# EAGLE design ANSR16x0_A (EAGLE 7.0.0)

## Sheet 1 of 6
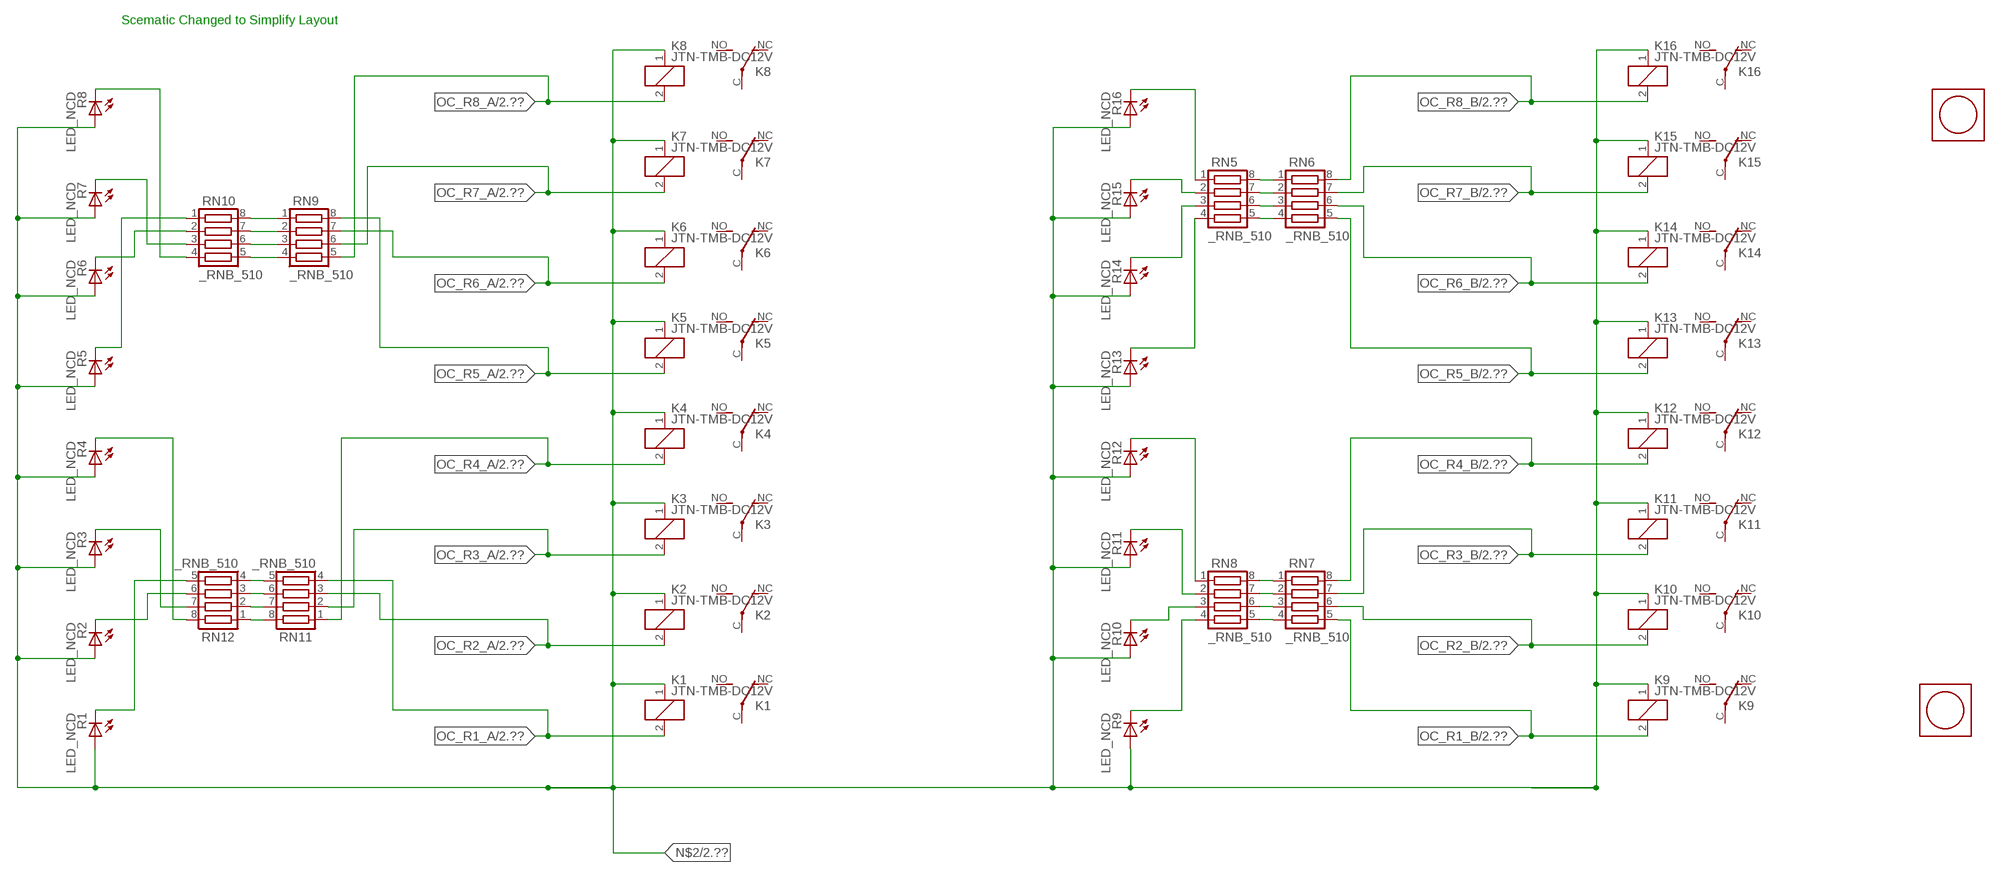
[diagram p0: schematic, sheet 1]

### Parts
K1  JTN-TMB-DC12V  [JT-TMB]
K2  JTN-TMB-DC12V  [JT-TMB]
K3  JTN-TMB-DC12V  [JT-TMB]
K4  JTN-TMB-DC12V  [JT-TMB]
K5  JTN-TMB-DC12V  [JT-TMB]
K6  JTN-TMB-DC12V  [JT-TMB]
K7  JTN-TMB-DC12V  [JT-TMB]
K8  JTN-TMB-DC12V  [JT-TMB]
K9  JTN-TMB-DC12V  [JT-TMB]
K10  JTN-TMB-DC12V  [JT-TMB]
K11  JTN-TMB-DC12V  [JT-TMB]
K12  JTN-TMB-DC12V  [JT-TMB]
K13  JTN-TMB-DC12V  [JT-TMB]
K14  JTN-TMB-DC12V  [JT-TMB]
K15  JTN-TMB-DC12V  [JT-TMB]
K16  JTN-TMB-DC12V  [JT-TMB]
R1  LED_NCD  [CHIPLED_0603]
R2  LED_NCD  [CHIPLED_0603]
R3  LED_NCD  [CHIPLED_0603]
R4  LED_NCD  [CHIPLED_0603]
R5  LED_NCD  [CHIPLED_0603]
R6  LED_NCD  [CHIPLED_0603]
R7  LED_NCD  [CHIPLED_0603]
R8  LED_NCD  [CHIPLED_0603]
R9  LED_NCD  [CHIPLED_0603]
R10  LED_NCD  [CHIPLED_0603]
R11  LED_NCD  [CHIPLED_0603]
R12  LED_NCD  [CHIPLED_0603]
R13  LED_NCD  [CHIPLED_0603]
R14  LED_NCD  [CHIPLED_0603]
R15  LED_NCD  [CHIPLED_0603]
R16  LED_NCD  [CHIPLED_0603]
RN5  _RNB_510  [RNB]
RN6  _RNB_510  [RNB]
RN7  _RNB_510  [RNB]
RN8  _RNB_510  [RNB]
RN9  _RNB_510  [RNB]
RN10  _RNB_510  [RNB]
RN11  _RNB_510  [RNB]
RN12  _RNB_510  [RNB]
U$1  PCB_MOUNTING_HOLE  [PCB_MOUNTING_HOLE]
U$3  PCB_MOUNTING_HOLE  [PCB_MOUNTING_HOLE]

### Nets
N$2: K1.1(C1) K2.1(C1) K3.1(C1) K4.1(C1) K5.1(C1) K6.1(C1) K7.1(C1) K8.1(C1) K9.1(C1) K10.1(C1) K11.1(C1) K12.1(C1) K13.1(C1) K14.1(C1) K15.1(C1) K16.1(C1) R1.A R2.A R3.A R4.A R5.A R6.A R7.A R8.A R9.A R10.A R11.A R12.A R13.A R14.A R15.A R16.A ; also sheet 2
N$441: R16.C RN5.1
N$442: RN7.2 RN8.7
N$443: RN7.3 RN8.6
N$444: RN7.4 RN8.5
N$445: R15.C RN5.2
N$447: R13.C RN5.4
N$448: RN5.5 RN6.4
N$449: RN7.1 RN8.8
N$450: R12.C RN8.1
N$451: RN5.6 RN6.3
N$452: R11.C RN8.2
N$453: RN5.7 RN6.2
N$454: RN5.8 RN6.1
N$458: R14.C RN5.3
N$459: R10.C RN8.3
N$463: RN11.5 RN12.4
N$470: R9.C RN8.4
N$473: R1.C RN12.5
N$474: RN11.6 RN12.3
N$475: R2.C RN12.6
N$476: R3.C RN12.7
N$477: RN9.4 RN10.5
N$478: RN9.3 RN10.6
N$479: RN9.2 RN10.7
N$480: RN9.1 RN10.8
N$481: RN11.7 RN12.2
N$482: R5.C RN10.1
N$483: R4.C RN12.8
N$484: R7.C RN10.3
N$485: R8.C RN10.4
N$486: R6.C RN10.2
N$500: RN11.8 RN12.1
OC_R1_A: K1.2(C2) RN11.4 ; also sheet 2
OC_R1_B: K9.2(C2) RN7.5 ; also sheet 2
OC_R2_A: K2.2(C2) RN11.3 ; also sheet 2
OC_R2_B: K10.2(C2) RN7.6 ; also sheet 2
OC_R3_A: K3.2(C2) RN11.2 ; also sheet 2
OC_R3_B: K11.2(C2) RN7.7 ; also sheet 2
OC_R4_A: K4.2(C2) RN11.1 ; also sheet 2
OC_R4_B: K12.2(C2) RN7.8 ; also sheet 2
OC_R5_A: K5.2(C2) RN9.8 ; also sheet 2
OC_R5_B: K13.2(C2) RN6.5 ; also sheet 2
OC_R6_A: K6.2(C2) RN9.7 ; also sheet 2
OC_R6_B: K14.2(C2) RN6.6 ; also sheet 2
OC_R7_A: K7.2(C2) RN9.6 ; also sheet 2
OC_R7_B: K15.2(C2) RN6.7 ; also sheet 2
OC_R8_A: K8.2(C2) RN9.5 ; also sheet 2
OC_R8_B: K16.2(C2) RN6.8 ; also sheet 2
Unconnected: K1.C(COM) K1.NC K1.NO K2.C(COM) K2.NC K2.NO K3.C(COM) K3.NC K3.NO K4.C(COM) K4.NC K4.NO K5.C(COM) K5.NC K5.NO K6.C(COM) K6.NC K6.NO K7.C(COM) K7.NC K7.NO K8.C(COM) K8.NC K8.NO K9.C(COM) K9.NC K9.NO K10.C(COM) K10.NC K10.NO K11.C(COM) K11.NC K11.NO K12.C(COM) K12.NC K12.NO K13.C(COM) K13.NC K13.NO K14.C(COM) K14.NC K14.NO K15.C(COM) K15.NC K15.NO K16.C(COM) K16.NC K16.NO

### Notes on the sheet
- Scematic Changed to Simplify Layout

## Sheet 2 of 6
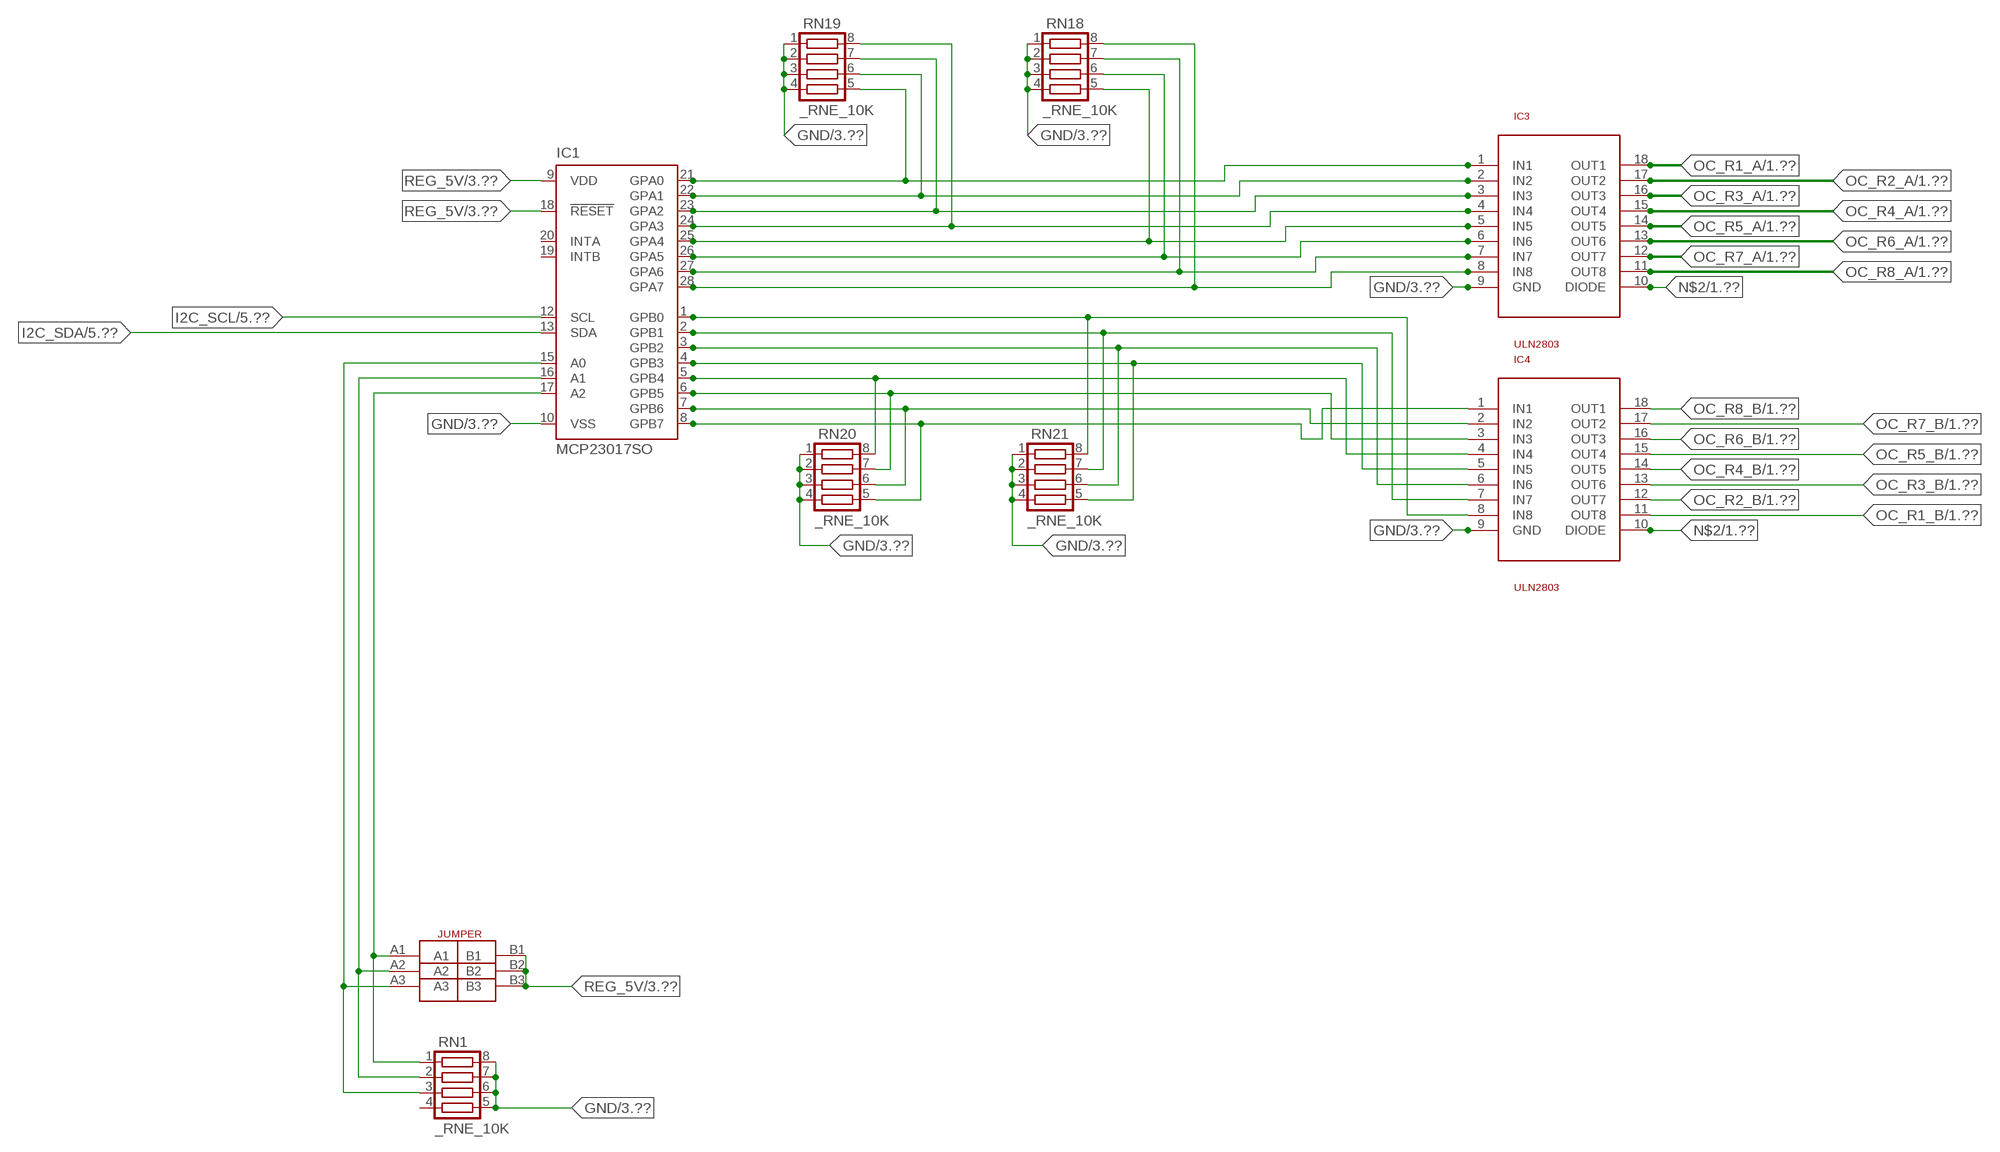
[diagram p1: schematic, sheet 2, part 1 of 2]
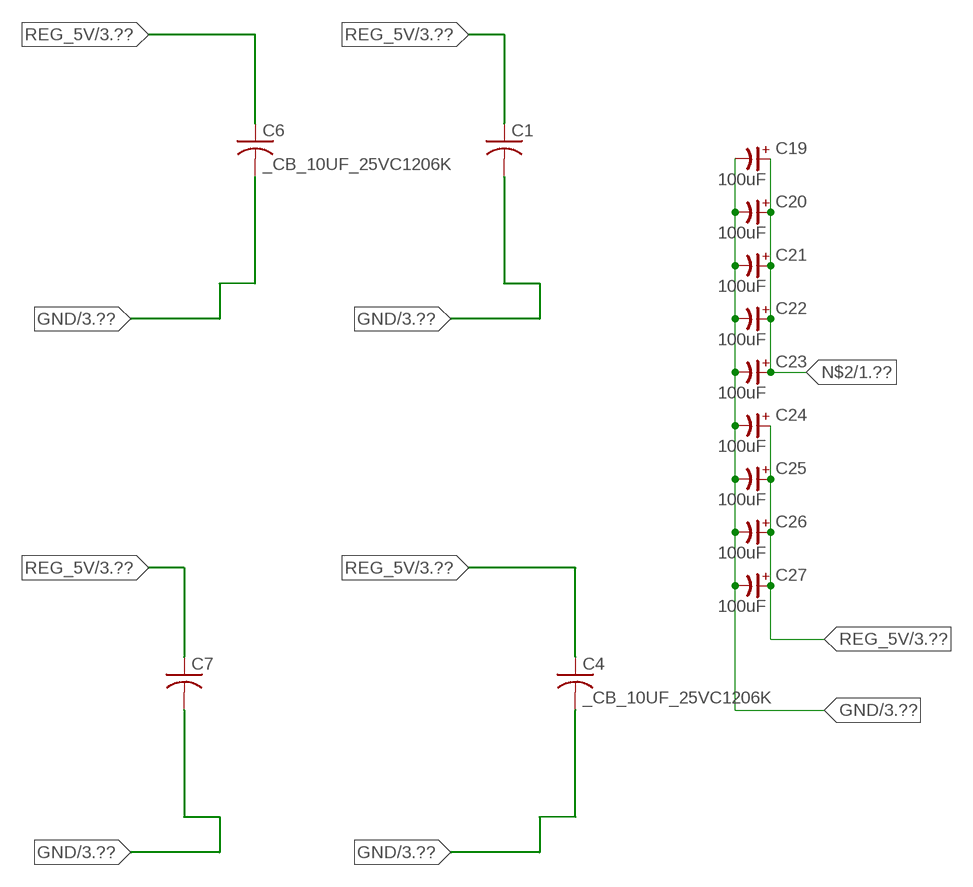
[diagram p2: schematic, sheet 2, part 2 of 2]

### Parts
C1  _CA_.10UF_50VC1206K  [_CA_.1UF_50V]
C4  _CB_10UF_25VC1206K  [_CB_10UF_25V]
C6  _CB_10UF_25VC1206K  [_CB_10UF_25V]
C7  _CA_.10UF_50VC1206K  [_CA_.1UF_50V]
C19  100uF  CP-E-025X060  [E-025X060]
C20  100uF  CP-E-025X060  [E-025X060]
C21  100uF  CP-E-025X060  [E-025X060]
C22  100uF  CP-E-025X060  [E-025X060]
C23  100uF  CP-E-025X060  [E-025X060]
C24  100uF  CP-E-025X060  [E-025X060]
C25  100uF  CP-E-025X060  [E-025X060]
C26  100uF  CP-E-025X060  [E-025X060]
C27  100uF  CP-E-025X060  [E-025X060]
IC1  MCP23017SO  [SO28W]
IC3  ULN2803  [SO18L]
IC4  ULN2803  [SO18L]
JP1  JUMPER_3X2  [JUMPER_3X2]
RN1  _RNE_10K  [RNE]
RN18  _RNE_10K  [RNE]
RN19  _RNE_10K  [RNE]
RN20  _RNE_10K  [RNE]
RN21  _RNE_10K  [RNE]

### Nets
GND: C1.2 C4.2 C6.2 C7.2 C19.- C20.- C21.- C22.- C23.- C24.- C25.- C26.- C27.- IC1.10(VSS) IC3.9(GND) IC4.9(GND) RN1.5 RN1.6 RN1.7 RN1.8 RN18.1 RN18.2 RN18.3 RN18.4 RN19.1 RN19.2 RN19.3 RN19.4 RN20.1 RN20.2 RN20.3 RN20.4 RN21.1 RN21.2 RN21.3 RN21.4 ; also sheet 3,4,5,6
I2C_SCL: IC1.12(SCL) ; also sheet 5,6
I2C_SDA: IC1.13(SDA) ; also sheet 5,6
N$2: C19.+ C20.+ C21.+ C22.+ C23.+ IC3.10(DIODE) IC4.10(DIODE) ; also sheet 1
N$4: IC1.15(A0) JP1.A3 RN1.3
N$405: IC1.21(GPA0) IC3.1(IN1) RN19.5
N$406: IC1.25(GPA4) IC3.5(IN5) RN18.5
N$407: IC1.26(GPA5) IC3.6(IN6) RN18.6
N$408: IC1.16(A1) JP1.A2 RN1.2
N$409: IC1.22(GPA1) IC3.2(IN2) RN19.6
N$410: IC1.23(GPA2) IC3.3(IN3) RN19.7
N$411: IC1.24(GPA3) IC3.4(IN4) RN19.8
N$416: IC1.1(GPB0) IC4.8(IN8) RN21.8
N$417: IC1.2(GPB1) IC4.7(IN7) RN21.7
N$418: IC1.3(GPB2) IC4.6(IN6) RN21.6
N$419: IC1.4(GPB3) IC4.5(IN5) RN21.5
N$420: IC1.5(GPB4) IC4.4(IN4) RN20.8
N$421: IC1.6(GPB5) IC4.3(IN3) RN20.7
N$422: IC1.7(GPB6) IC4.2(IN2) RN20.6
N$423: IC1.8(GPB7) IC4.1(IN1) RN20.5
N$498: IC1.17(A2) JP1.A1 RN1.1
N$525: IC1.27(GPA6) IC3.7(IN7) RN18.7
N$526: IC1.28(GPA7) IC3.8(IN8) RN18.8
OC_R1_A: IC3.18(OUT1) ; also sheet 1
OC_R1_B: IC4.11(OUT8) ; also sheet 1
OC_R2_A: IC3.17(OUT2) ; also sheet 1
OC_R2_B: IC4.12(OUT7) ; also sheet 1
OC_R3_A: IC3.16(OUT3) ; also sheet 1
OC_R3_B: IC4.13(OUT6) ; also sheet 1
OC_R4_A: IC3.15(OUT4) ; also sheet 1
OC_R4_B: IC4.14(OUT5) ; also sheet 1
OC_R5_A: IC3.14(OUT5) ; also sheet 1
OC_R5_B: IC4.15(OUT4) ; also sheet 1
OC_R6_A: IC3.13(OUT6) ; also sheet 1
OC_R6_B: IC4.16(OUT3) ; also sheet 1
OC_R7_A: IC3.12(OUT7) ; also sheet 1
OC_R7_B: IC4.17(OUT2) ; also sheet 1
OC_R8_A: IC3.11(OUT8) ; also sheet 1
OC_R8_B: IC4.18(OUT1) ; also sheet 1
REG_5V: C1.1 C4.1 C6.1 C7.1 C24.+ C25.+ C26.+ C27.+ IC1.9(VDD) IC1.18(!RESET) JP1.B1 JP1.B2 JP1.B3 ; also sheet 3,4,5,6
Unconnected: IC1.19(INTB) IC1.20(INTA) RN1.4

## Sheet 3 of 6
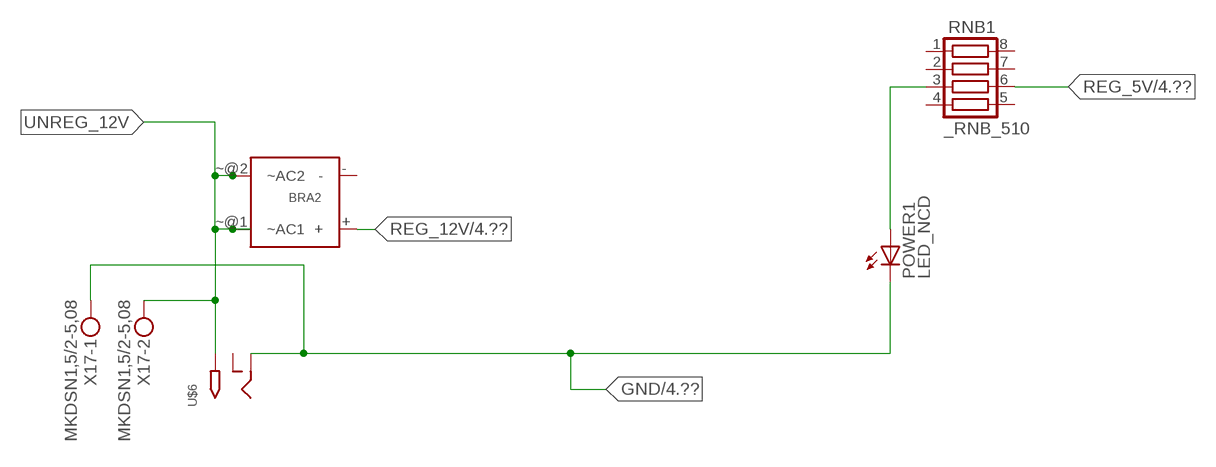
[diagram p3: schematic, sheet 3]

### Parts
BRA2  MB2S_  [MB2S]
POWER1  LED_NCD  [CHIPLED_0603]
RNB1  _RNB_510  [RNB]
U$6  2.1MMJACK  [PJ-102A]
X17  MKDSN1,5/2-5,08  [MKDSN1,5/2-5,08]

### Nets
GND: POWER1.C U$6.RING X17.1 ; also sheet 2,4,5,6
N$99: POWER1.A RNB1.3
REG_5V: RNB1.6 ; also sheet 2,4,5,6
REG_12V: BRA2.+ ; also sheet 4
UNREG_12V: BRA2.~@1(~AC1) BRA2.~@2(~AC2) U$6.TIP X17.2
Unconnected: BRA2.- RNB1.1 RNB1.2 RNB1.4 RNB1.5 RNB1.7 RNB1.8 U$6.RING_SW

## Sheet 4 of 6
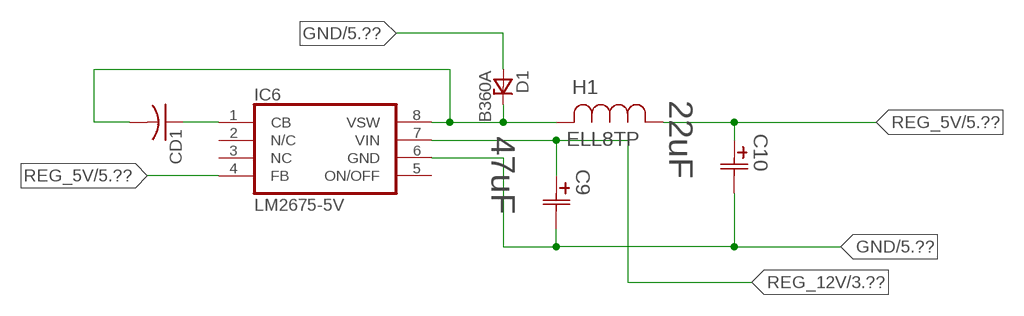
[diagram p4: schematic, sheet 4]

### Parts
C9  47uF  490-5463-6-NDCAP  [C2917(7343)-Y]
C10  22uF  490-5463-6-NDCAP  [C2917(7343)-Y]
CD1  _CD_10NF_50VC1206K  [_CD_10NF_50V]
D1  B360A  [DO214AC_ZENER]
H1  ELL8TP  [IND_ELL8TP]
IC6  LM2675-5V  LM2675  [SO-8]

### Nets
GND: C9.2(C2) C10.2(C2) D1.A IC6.6(GND) ; also sheet 2,3,5,6
N$100: CD1.2 D1.C H1.2 IC6.8(VSW)
N$101: CD1.1 IC6.1(CB)
REG_5V: C10.1(C1) H1.1 IC6.4(FB) ; also sheet 2,3,5,6
REG_12V: C9.1(C1) IC6.7(VIN) ; also sheet 3
Unconnected: IC6.2(N/C) IC6.5(ON/OFF)

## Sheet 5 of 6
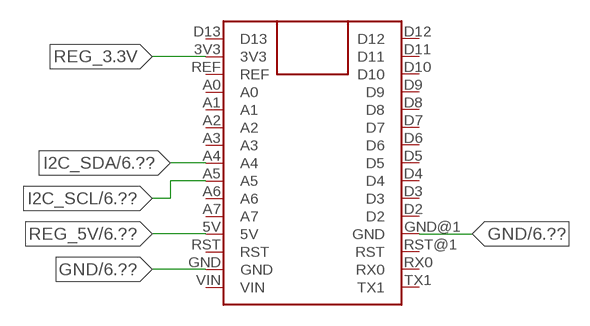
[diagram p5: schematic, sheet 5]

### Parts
FOR_NANO  ARDUINO_NANO  [ARDUINO_NANO]

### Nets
GND: FOR_NANO.GND FOR_NANO.GND@1(GND) ; also sheet 2,3,4,6
I2C_SCL: FOR_NANO.A5 ; also sheet 2,6
I2C_SDA: FOR_NANO.A4 ; also sheet 2,6
REG_3.3V: FOR_NANO.3V3
REG_5V: FOR_NANO.5V ; also sheet 2,3,4,6
Unconnected: FOR_NANO.A0 FOR_NANO.A1 FOR_NANO.A2 FOR_NANO.A3 FOR_NANO.A6 FOR_NANO.A7 FOR_NANO.D2 FOR_NANO.D3 FOR_NANO.D4 FOR_NANO.D5 FOR_NANO.D6 FOR_NANO.D7 FOR_NANO.D8 FOR_NANO.D9 FOR_NANO.D10 FOR_NANO.D11 FOR_NANO.D12 FOR_NANO.D13 FOR_NANO.REF FOR_NANO.RST FOR_NANO.RST@1(RST) FOR_NANO.RX0 FOR_NANO.TX1 FOR_NANO.VIN

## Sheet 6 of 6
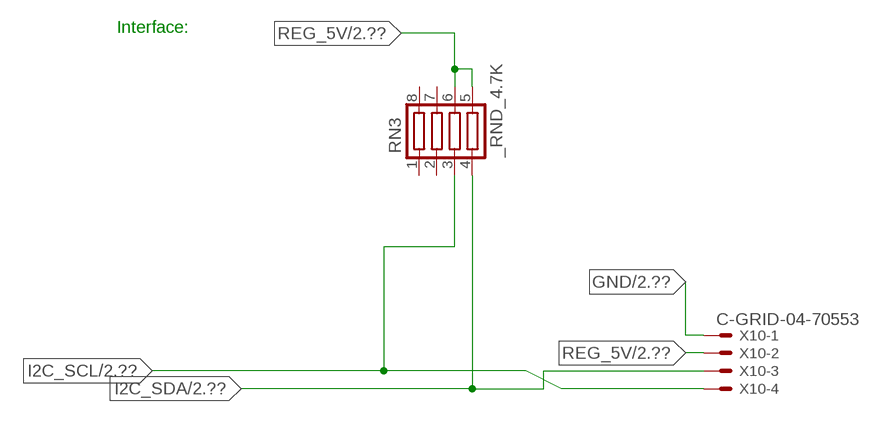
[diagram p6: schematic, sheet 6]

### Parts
RN3  _RND_4.7K  [RND]
X10  C-GRID-04-70553  [70553-04]

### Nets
GND: X10.1 ; also sheet 2,3,4,5
I2C_SCL: RN3.3 X10.4 ; also sheet 2,5
I2C_SDA: RN3.4 X10.3 ; also sheet 2,5
REG_5V: RN3.5 RN3.6 X10.2 ; also sheet 2,3,4,5
Unconnected: RN3.1 RN3.2 RN3.7 RN3.8

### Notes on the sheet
- Interface:

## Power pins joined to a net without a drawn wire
NC: IC6.3(NC)

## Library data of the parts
BRA2 = NCD_ULTIMATE_LIBRARY:MB2S: Bridge Rectifier BRA MB2S 200V 500ma Digikey MB2S-TPMSTR-ND/MB2S-TP
C1 C7 = NCD_ULTIMATE_LIBRARY:_CA_.10UF_50V: Capacitor .1uF SMT
C4 C6 = NCD_ULTIMATE_LIBRARY:_CB_10UF_25V: Capacitor 10uF SMT
C9 C10 = NCD_ULTIMATE_bhaskar:490-5463-6-ND: NCD CAP
C19-C27 = NCD_ULTIMATE_LIBRARY:CP-: Capacitors All Kinds POLARIZED CAP
CD1 = NCD_ULTIMATE_LIBRARY:_CD_10NF_50V: Capacitor 10nF SMT
D1 = NCD_ULTIMATE_bhaskar:B360A: NCD DIODE B350A/B360A
FOR_NANO = NCD_ULTIMATE_CONNECTORS:ARDUINO_NANO
H1 = NCD_ULTIMATE_bhaskar:ELL8TP: NCD coil
IC1 = NCD_ULTIMATE_LIBRARY:MCP23017: Semiconductor Port Expander I/O 16-Bit I2C http://ww1.microchip.com/downloads/en/DeviceDoc/21952a.pdf Source: http://ww1.microchip.com/downloads/en/DeviceDoc/21952a.pdf
IC3 IC4 = NCD_ULTIMATE_LIBRARY:ULN2803: Semiconductor 8 O.C. N-Channel Transistor Driver Digikey ULN2803AFWGCELTR-ND/ULN2803AFWG,C,EL
IC6 = NCD_ULTIMATE_bhaskar:LM2675: LM2675 NCD http://www.ti.com/lit/ds/symlink/lm2675.pdf
JP1 = NCD_ULTIMATE_CONNECTORS:JUMPER_3X2
K1-K16 = NCD_ULTIMATE_LIBRARY:JT?-*: RELAY COMPACT ECONOMICAL 30 AMP. RELAY NAiS Source: http://www.mew-europe.com/.. en_ds_61212_0000.pdf
POWER1 R1-R16 = NCD_ULTIMATE_bhaskar:LED_NCD
RN1 RN18-RN21 = NCD_ULTIMATE_LIBRARY:_RNE_10K: Resistor Array RNE SMT 10K x 4 Single Resistor Source: http://www.ctscorp.com/components/Datasheets/CTSChipArrayDs.pdf Digikey 742C083103JPTR-ND/742C083103JP; OC_FARNELL: unknown; OC_NEWARK: unknown
RN3 = NCD_ULTIMATE_LIBRARY:_RND_4.7K: Resistor Array RND SMT 4.7K x 4 Single Resistor Source: http://www.ctscorp.com/components/Datasheets/CTSChipArrayDs.pdf Digikey 742C083472JPTR-ND/742C083472JP; OC_FARNELL: unknown; OC_NEWARK: unknown
RN5-RN12 RNB1 = NCD_ULTIMATE_LIBRARY:_RNB_510: Resistor Array RNB SMT 510 x 4 Single Resistor Source: http://www.ctscorp.com/components/Datasheets/CTSChipArrayDs.pdf Digikey 742C083511JPTR-ND/ 742C083511JP; OC_FARNELL: unknown; OC_NEWARK: unknown
U$1 U$3 = NCD_ULTIMATE_CONNECTORS:PCB_MOUNTING_HOLE
U$6 = NCD_ULTIMATE_CONNECTORS:2.1MMJACK: 2.1mm x 5.5mm DC jack with internal switch. Digikey part #PJ-102A, 4UCON part #05537 By microbuilder.eu
X10 = NCD_ULTIMATE_CONNECTORS:C-GRID-04: CONNECTOR 4-Pos I2C wire to board 2.54 mm (0.100") pitch header Digikey WM1342-ND/0015912045; OC_FARNELL: unknown; OC_NEWARK: unknown
X17 = NCD_ULTIMATE_CONNECTORS:MKDSN1,5/2-5,08: MKDSN 1,5/ 2-5,08 Printklemme

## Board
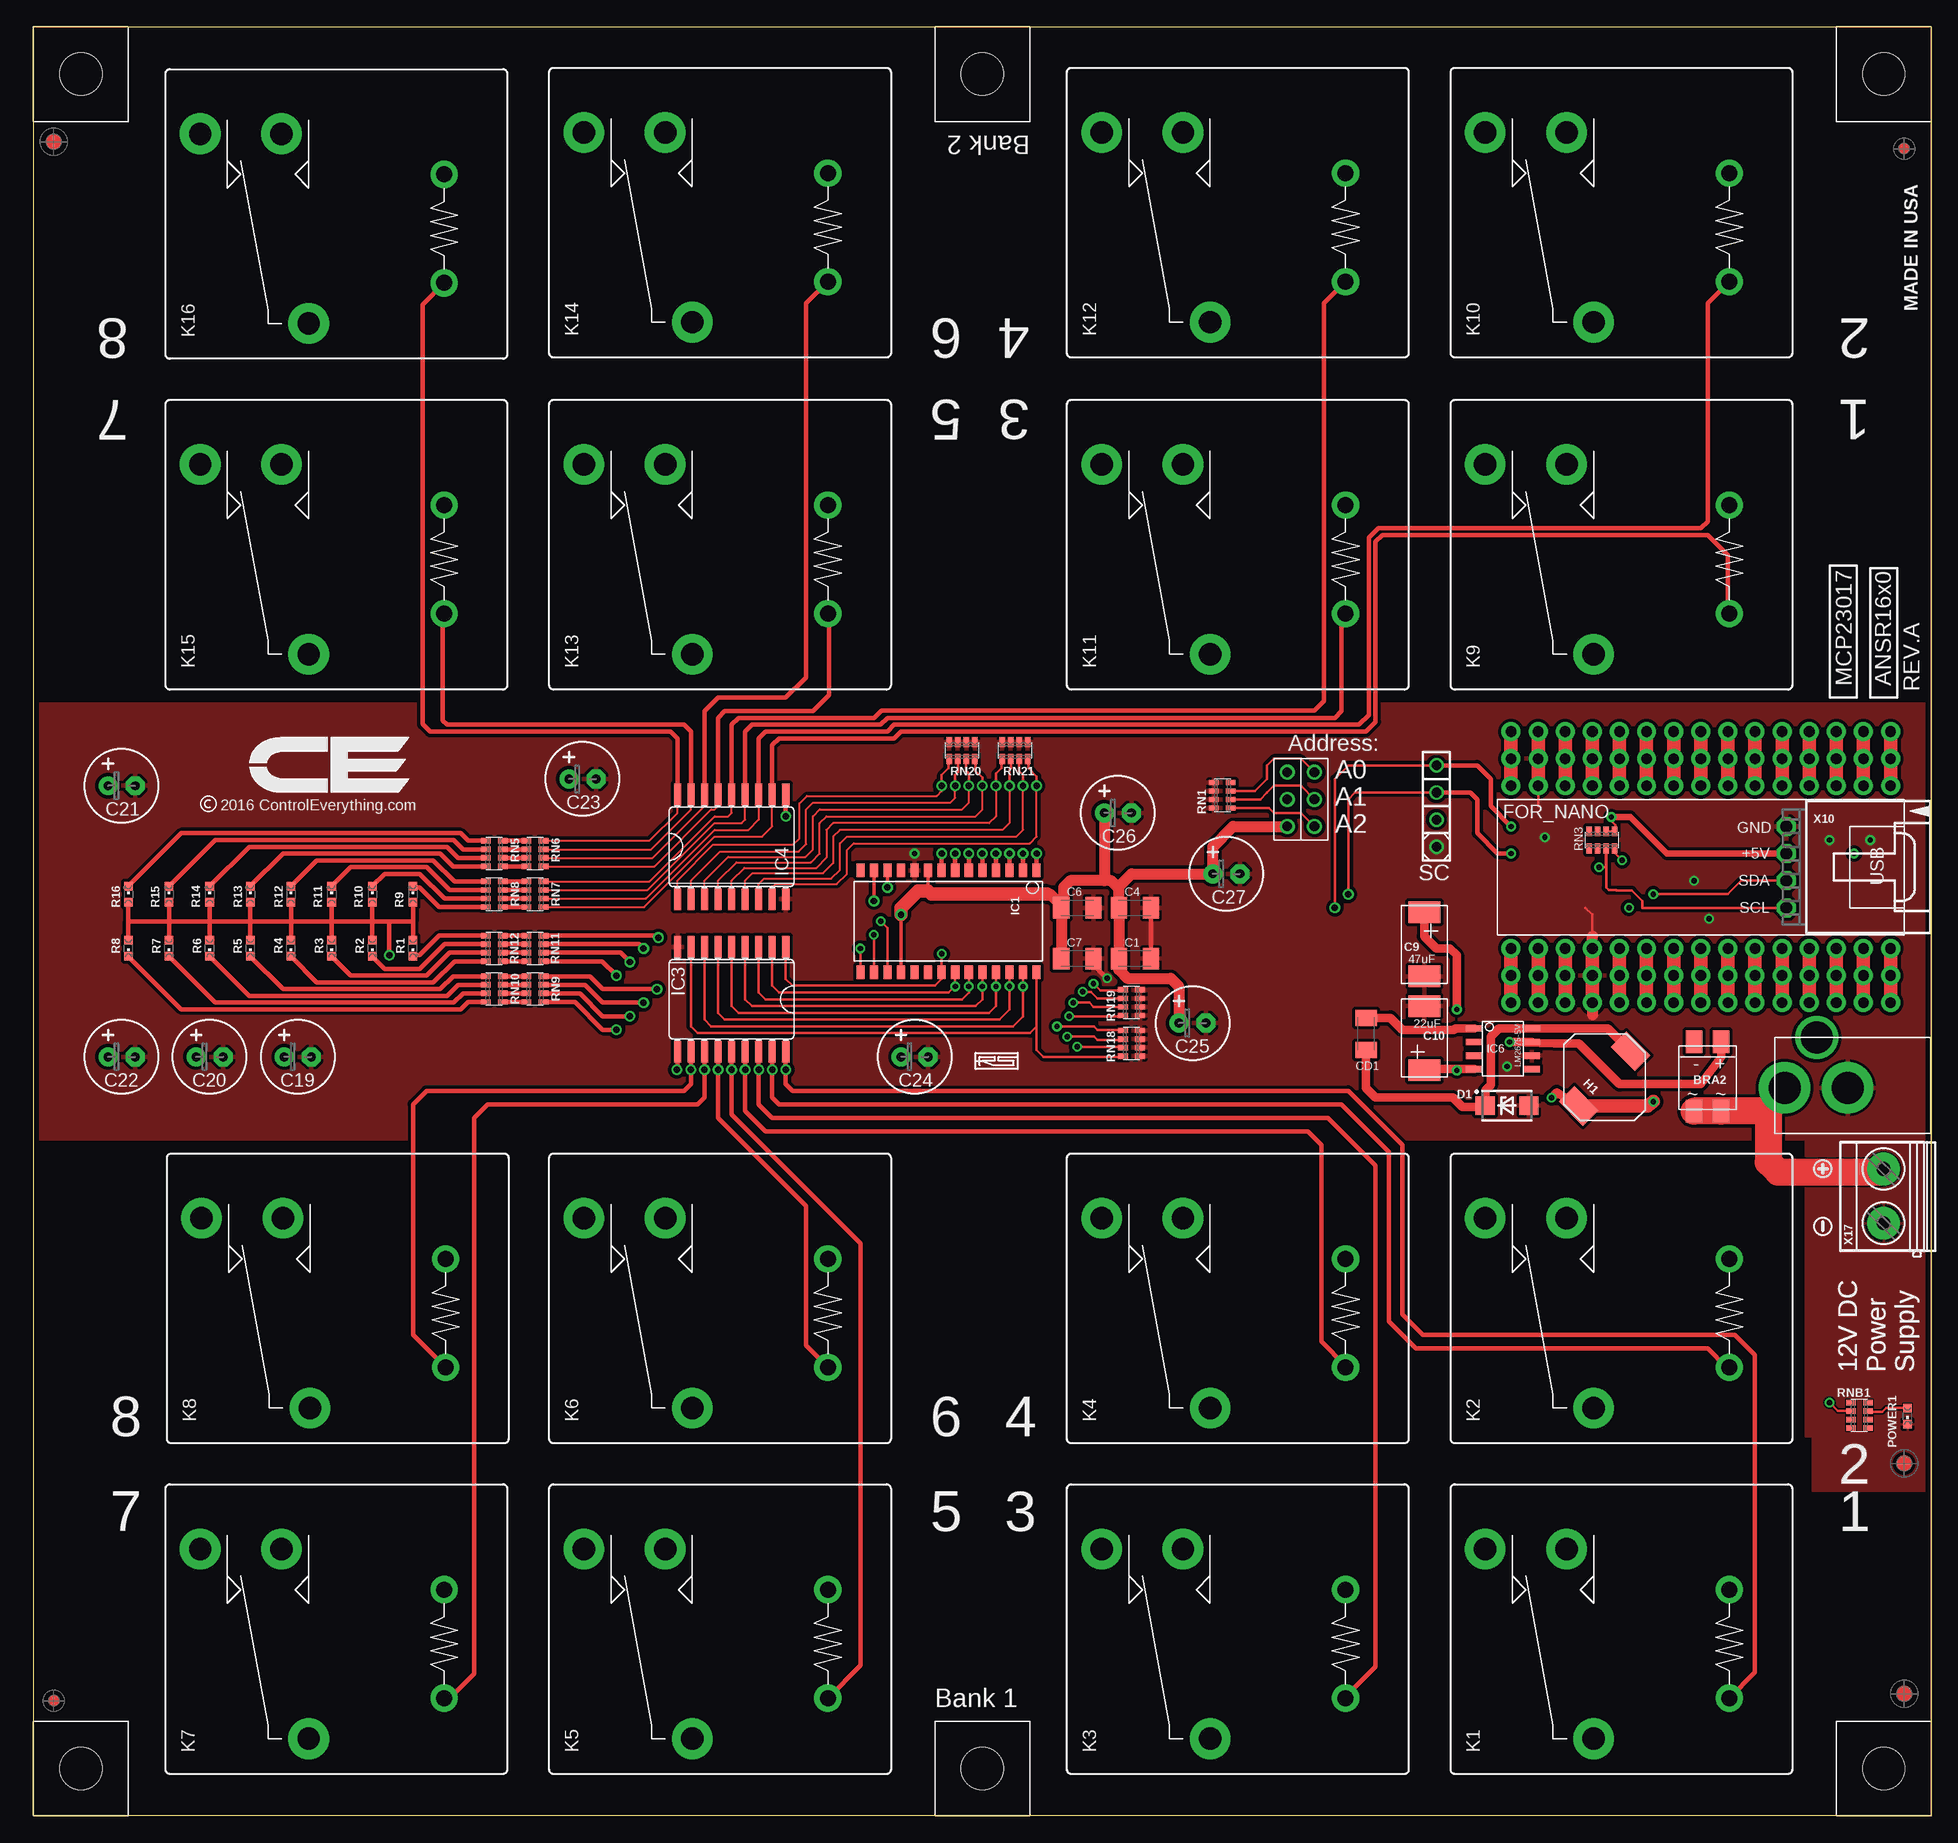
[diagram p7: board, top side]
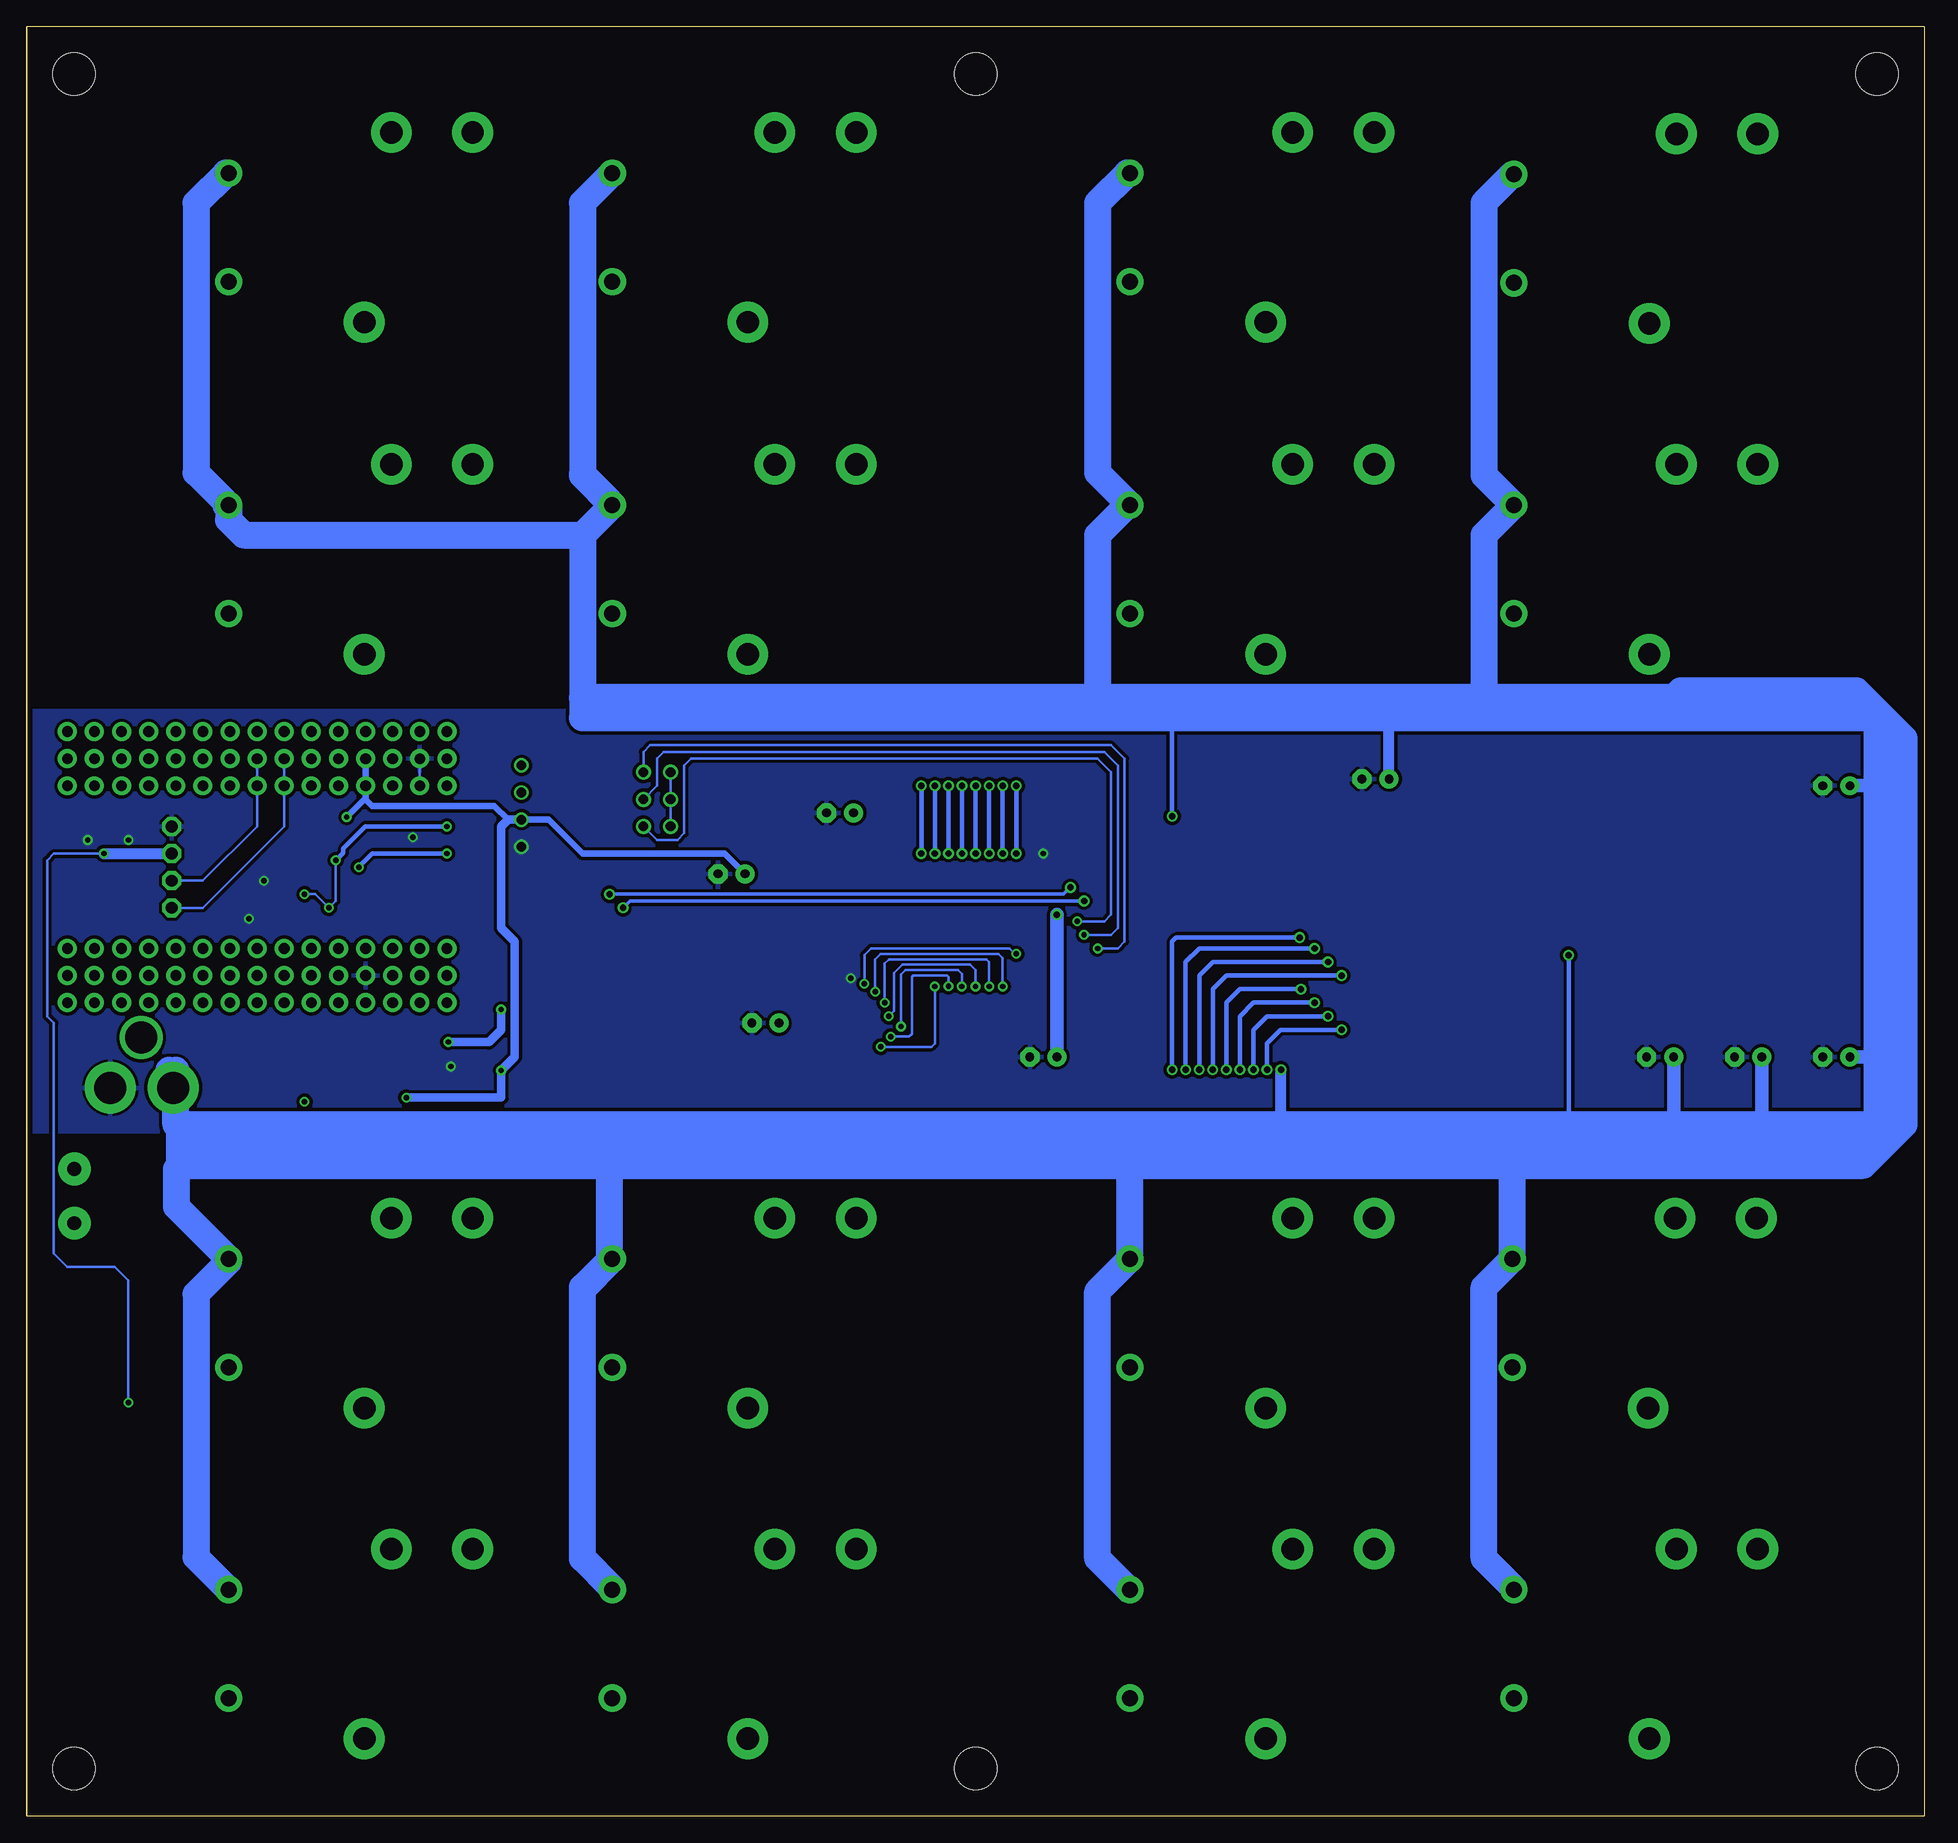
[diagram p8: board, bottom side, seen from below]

Size 177.8 x 167.65 mm. Coordinates in mm from the lower left corner, seen from the top.
Outline: 177.78,0 177.78,167.65 0,167.65 0,0.01 177.8,0.01 177.8,167.65
Outline: 177.78,101.61 177.78,21.59
Outline: 177.78,102.88 177.78,22.22
Outline: 177.8,102.88 177.8,45.1
Copper layers (1*16): Top 0.035mm / dielectric 1.5mm / Bottom 0.035mm
Design rules "default *": minimum track width 6mil, minimum drill 12mil, track to track 5mil, track to pad 5mil, pad to pad 5mil, via to via 5mil, smd to smd 5mil, copper to edge 20mil, drill to drill 8mil, minimum pad ring 10mil, minimum via ring 8mil, stop-mask expansion 4mil, vias tented up to drill 0mil, thermal gap 10mil

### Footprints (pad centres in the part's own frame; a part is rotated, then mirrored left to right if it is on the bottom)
MB2S = smd 1.55 x 2.1: + 0,-6.5; - 2.54,-6.5; ~@1 0,0; ~@2 2.54,0
_CA_.1UF_50V = smd 1.5 x 2: 1 -1.5,0; 2 1.5,0
_CB_10UF_25V = smd 1.5 x 2: 1 -1.5,0; 2 1.5,0
C2917(7343)-Y = smd 2 x 3: 1 -3,0; 2 3,0
E-025X060 = drill 0.813 pad 1.778: + -1.27,0 | drill 0.813 pad 1.778 octagon: - 1.27,0
_CD_10NF_50V = smd 1.5 x 2: 1 -1.5,0; 2 1.5,0
DO214AC_ZENER = smd 1.8 x 1.7: A 2.05,0; C -2.05,0
ARDUINO_NANO = drill 1 pad 1.778: 3V1 -2.54,-2.54; 3V3 0,-2.54; 5V 0,-27.94; 5V1 -2.54,-27.94; A0 0,-7.62; A1 0,-10.16; A2 0,-12.7; A3 0,-15.24; A4 0,-17.78; A5 0,-20.32; A6 0,-22.86; A7 0,-25.4; A8 -2.54,-7.62; A9 -2.54,-10.16; A10 -2.54,-12.7; A11 -2.54,-15.24; A12 -2.54,-17.78; A13 -2.54,-20.32; A14 -2.54,-22.86; A15 -2.54,-25.4; D1 -2.54,0; D2 20.32,-25.4; D3 20.32,-22.86; D4 20.32,-20.32; D5 20.32,-17.78; D6 20.32,-15.24; D7 20.32,-12.7; D8 20.32,-10.16; D9 20.32,-7.62; D10 20.32,-5.08; D11 20.32,-2.54; D12 20.32,0; D13 0,0; D14 22.86,0; D15 22.86,-2.54; D16 22.86,-5.08; D17 22.86,-7.62; D18 22.86,-10.16; D19 22.86,-12.7; D20 22.86,-15.24; D21 22.86,-17.78; D22 22.86,-20.32; D23 22.86,-22.86; D24 22.86,-25.4; GND 0,-33.02; GND1 -2.54,-33.02; GND@1 20.32,-27.94; GND@2 22.86,-27.94; P$16 2.54,0; P$17 2.54,-2.54; P$18 2.54,-5.08; P$19 2.54,-7.62; P$20 2.54,-10.16; P$21 2.54,-12.7; P$22 2.54,-15.24; P$23 2.54,-17.78; P$24 2.54,-20.32; P$25 2.54,-22.86; P$26 2.54,-25.4; P$27 2.54,-27.94; P$28 2.54,-30.48; P$29 2.54,-33.02; P$30 2.54,-35.56; P$31 17.78,0; P$32 17.78,-2.54; P$33 17.78,-5.08; P$34 17.78,-7.62; P$35 17.78,-10.16; P$36 17.78,-12.7; P$37 17.78,-15.24; P$38 17.78,-17.78; P$39 17.78,-20.32; P$40 17.78,-22.86; P$41 17.78,-25.4; P$42 17.78,-27.94; P$43 17.78,-30.48; P$44 17.78,-33.02; P$45 17.78,-35.56; REF 0,-5.08; REF1 -2.54,-5.08; RST 0,-30.48; RST1 -2.54,-30.48; RST@1 20.32,-30.48; RST@2 22.86,-30.48; RX0 20.32,-33.02; RX1 22.86,-33.02; TX1 20.32,-35.56; TX2 22.86,-35.56; VIN 0,-35.56; VIN1 -2.54,-35.56
IND_ELL8TP = smd 2.054 x 3.2 rotated 45: 1 -2.442,-2.696; 2 2.442,2.442
SO28W = smd 0.762 x 1.27: 1 -7.62,-4.78; 2 -6.35,-4.78; 3 -5.08,-4.78; 4 -3.81,-4.78; 5 -2.54,-4.78; 6 -1.27,-4.78; 7 0,-4.78; 8 1.27,-4.78; 9 2.54,-4.78; 10 3.81,-4.78; 11 5.08,-4.78; 12 6.35,-4.78; 13 7.62,-4.78; 14 8.89,-4.78; 15 8.89,4.78; 16 7.62,4.78; 17 6.35,4.78; 18 5.08,4.78; 19 3.81,4.78; 20 2.54,4.78; 21 1.27,4.78; 22 0,4.78; 23 -1.27,4.78; 24 -2.54,4.78; 25 -3.81,4.78; 26 -5.08,4.78; 27 -6.35,4.78; 28 -7.62,4.78
SO18L = smd 0.66 x 2.032: 1 -5.08,-4.902; 2 -3.81,-4.902; 3 -2.54,-4.902; 4 -1.27,-4.902; 5 0,-4.902; 6 1.27,-4.902; 7 2.54,-4.902; 8 3.81,-4.902; 9 5.08,-4.902; 10 5.08,4.902; 11 3.81,4.902; 12 2.54,4.902; 13 1.27,4.902; 14 0,4.902; 15 -1.27,4.902; 16 -2.54,4.902; 17 -3.81,4.902; 18 -5.08,4.902
SO-8 = smd 0.6 x 1.55: 1 -1.905,-2.69; 2 -0.635,-2.69; 3 0.635,-2.69; 4 1.905,-2.69; 5 1.905,2.71; 6 0.635,2.71; 7 -0.635,2.71; 8 -1.905,2.71
JUMPER_3X2 = drill 0.9: A1 0,5.08; A2 0,2.54; A3 0,0; B1 2.54,5.08; B2 2.54,2.54; B3 2.54,0
JT-TMB = drill 1.5 pad 2.54: 1 5.08,0; 2 -5.08,0 | drill 2.1 pad 3.81: C -8.89,12.7; NC 8.89,22.86; NO 8.89,15.24
CHIPLED_0603 = smd 0.8 x 0.8: A 0,-0.75; C 0,0.75
RNE = smd 0.5 x 0.9: 1 -1.2,-0.8; 2 -0.4,-0.8; 3 0.4,-0.8; 4 1.2,-0.8; 5 1.2,0.8; 6 0.4,0.8; 7 -0.4,0.8; 8 -1.2,0.8
RND = smd 0.5 x 0.9: 1 -1.2,-0.8; 2 -0.4,-0.8; 3 0.4,-0.8; 4 1.2,-0.8; 5 1.2,0.8; 6 0.4,0.8; 7 -0.4,0.8; 8 -1.2,0.8
RNB = smd 0.5 x 0.9: 1 -1.2,-0.8; 2 -0.4,-0.8; 3 0.4,-0.8; 4 1.2,-0.8; 5 1.2,0.8; 6 0.4,0.8; 7 -0.4,0.8; 8 -1.2,0.8
PCB_MOUNTING_HOLE = hole 3.962: 4.445,4.445
PJ-102A = drill 3 pad 4.8: RING 0.1,-3.39; TIP 0.1,-9.29 | drill 3 pad 3.251: RING_SW -4.6,-6.29
70553-04 = drill 1.1 pad 1.778 octagon: 1 -3.81,-7.62; 2 -1.27,-7.62; 3 1.27,-7.62; 4 3.81,-7.62
MKDSN1,5/2-5,08 = drill 1.3 pad 3.048: 1 -2.561,0.025; 2 2.519,0.025

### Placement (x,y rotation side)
BRA2  158.12,66.05 180 top
C1  103.19,80.34 0 top
C4  103.19,85.1 0 top
C6  97.79,85.1 0 top
C7  97.79,80.34 0 top
C9  130.3,81.67 270 top
C10  130.3,72.89 90 top
C19  24.77,71.13 0 top
C20  16.51,71.13 0 top
C21  8.26,96.53 0 top
C22  8.26,71.13 0 top
C23  51.44,97.17 0 top
C24  82.55,71.13 0 top
C25  108.58,74.31 0 top
C26  101.6,93.99 0 top
C27  111.76,88.28 0 top
CD1  124.84,73.29 270 top
D1  138.05,66.56 0 top
FOR_NANO  173.99,99.07 270 top
H1  147.19,69.23 0 top
IC1  86.36,83.83 180 top
IC3  65.41,76.53 180 top
IC4  65.41,90.82 0 top
IC6  137.67,71.89 270 top
JP1  120.02,97.8 180 top
K1  158.88,16.14 90 top
K2  158.88,47.13 90 top
K3  122.94,16.14 90 top
K4  122.94,47.13 90 top
K5  74.42,16.14 90 top
K6  74.42,47.13 90 top
K7  38.48,16.14 90 top
K8  38.61,47.13 90 top
K9  158.88,117.74 90 top
K10  158.88,148.86 90 top
K11  122.94,117.74 90 top
K12  122.94,148.86 90 top
K13  74.42,117.74 90 top
K14  74.42,148.86 90 top
K15  38.48,117.74 90 top
K16  38.48,148.73 90 top
POWER1  175.58,37.48 180 top
R1  35.56,81.29 180 top
R2  31.75,81.29 180 top
R3  27.94,81.29 180 top
R4  24.13,81.29 180 top
R5  20.32,81.29 180 top
R6  16.51,81.29 180 top
R7  12.7,81.29 180 top
R8  8.89,81.29 180 top
R9  35.56,86.37 0 top
R10  31.75,86.37 0 top
R11  27.94,86.37 0 top
R12  24.13,86.37 0 top
R13  20.32,86.37 0 top
R14  16.51,86.37 0 top
R15  12.7,86.37 0 top
R16  8.89,86.37 0 top
RN1  111.38,95.64 90 top
RN3  146.94,91.45 0 top
RN5  43.18,90.18 270 top
RN6  46.99,90.18 270 top
RN7  46.99,86.37 270 top
RN8  43.18,86.37 270 top
RN9  46.99,77.48 270 top
RN10  43.18,77.48 270 top
RN11  46.99,81.29 90 top
RN12  43.18,81.29 90 top
RN18  102.87,72.4 90 top
RN19  102.87,76.21 90 top
RN20  87,99.83 180 top
RN21  91.95,99.83 180 top
RNB1  171.07,37.54 90 top
U$1  93.34,158.76 90 top
U$3  177.8,158.76 90 top
U$5  PCB_MOUNTING_HOLE  [PCB_MOUNTING_HOLE]  0,8.9 270 top
U$6  173.35,68.34 270 top
U$7  [ICON_MINUS]  167.64,55.26 90 top
U$8  [ICON_PLUS]  167.64,60.66 0 top
U$9  PCB_MOUNTING_HOLE  [PCB_MOUNTING_HOLE]  8.89,158.76 90 top
U$10  PCB_MOUNTING_HOLE  [PCB_MOUNTING_HOLE]  84.45,8.9 270 top
U$11  PCB_MOUNTING_HOLE  [PCB_MOUNTING_HOLE]  168.91,8.9 270 top
U$12  PCB_MOUNTING_HOLE  [PCB_MOUNTING_HOLE]  0,8.9 270 top
U$13  [VISION_REF15]  175.26,33.03 90 top
U$15  [VISION_REF15]  175.26,11.44 90 top
U$17  [ICON_MINUS]  167.64,55.26 90 top
U$18  [VISION_REF10]  175.26,156.22 90 top
U$19  [ICON_PLUS]  167.64,60.66 0 top
U$21  [ICON_USA]  176.53,140.98 90 top
U$22  [ICON_MINUS]  167.64,55.26 90 top
U$23  [VISION_REF15]  1.91,156.86 90 top
U$24  [ICON_PLUS]  167.64,60.66 0 top
U$28  [VISION_REF10]  1.91,10.81 90 top
X10  171.83,88.91 270 top
X17  173.35,58.12 90 top

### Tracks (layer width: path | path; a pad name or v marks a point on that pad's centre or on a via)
GND  (via drill 0.5, 0.9)
  Top 0.254: 146.05,82.44 146.05,84.47 145.41,85.1 | FOR_NANO.GND@1 146.05,77.48 | 140.97,101.61 140.97,94.63
  Top 0.406: C1.2 C4.2 | v100.58,78.5 99.69,79.39 99.69,79.93 C7.2
  Top 1.016: X10.1 164.06,92.72 | 146.05,75.07 146.05,81.29 146.05,82.44
  Bottom 0.254: 140.97,96.53 FOR_NANO.GND
  other vias: 82.55,90.18 131.44,90.82 168.28,91.45 141.6,91.71 172.09,91.45 155.57,87.64 156.97,84.09 138.05,70.24
  pour Top (isolate 0.305): -5.71,63.51 -5.71,104.15 177.48,104.15 177.48,63.51
  pour Top: 177.48,51.45 166.05,51.45 166.05,63.51 177.48,63.51
  pour Bottom (isolate 0.305): -3.17,103.52 177.16,103.52 177.16,64.15 -3.17,64.15
  pour Top: 177.48,35.57 166.05,35.57 166.05,63.51 177.48,63.51
  pour Top: 177.48,30.49 166.69,30.49 166.69,63.51 177.48,63.51
I2C_SCL  (via drill 0.5, 0.6, 0.9)
  Top 0.254: v131.44,95.9 123.83,95.9 123.19,95.26 v123.19,86.37 | X10.4 150.75,85.1 150.75,85.74 149.75,86.74 148.32,86.74 148.3,86.75 147.57,86.75 147.34,86.99 RN3.3 147.32,90.63 147.32,88.91 v146.69,88.91
  Top 0.305: v80.01,87.01 IC1.12
  Top 0.406: v131.44,95.9 134.62,95.9 135.25,95.26 135.25,92.09 137.16,90.18 v138.43,90.18
  Bottom 0.254: FOR_NANO.A5 153.67,92.72 161.29,85.1 X10.4
  Bottom 0.305: v123.19,86.37 80.64,86.37 v80.01,87.01
  Bottom 0.406: v138.43,90.18 145.41,90.18 v146.69,88.91
I2C_SDA  (via drill 0.5, 0.6, 0.9)
  Top 0.254: v131.44,98.44 123.19,98.44 121.92,97.17 v121.92,85.1 | RN3.4 148.14,90.25 v148.84,89.55 | v149.47,85.09 v149.48,85.1 | X10.3 160.02,87.64 158.75,86.37 v151.76,86.37
  Top 0.305: v78.74,85.74 IC1.13
  Top 0.406: v131.44,98.44 135.25,98.44 136.53,97.17 136.53,94.63 v138.43,92.72
  Bottom 0.254: v148.84,89.55 148.84,85.74 v149.48,85.1 150.75,86.37 v151.76,86.37 | FOR_NANO.A4 156.21,92.72 161.29,87.64 X10.3
  Bottom 0.305: v78.74,85.74 121.28,85.74 v121.92,85.1
  Bottom 0.406: v138.43,92.72 146.07,92.72 RN3.4 148.14,90.25 v148.84,89.55
N$2  (via drill 0.6)
  Top 0.305: 35.56,83.83 R1.A
  Top 0.406: IC4.10 v70.48,93.67 | R8.A 8.89,83.83 | R15.A 12.7,83.83 | R6.A 16.51,83.83 | 20.32,83.83 R13.A | R4.A 24.13,83.83 | R3.A 27.94,83.83 | R2.A 31.75,83.83 | R16.A 8.89,83.83 | 8.89,83.83 12.7,83.83 | R7.A 12.7,83.83 | 12.7,83.83 16.51,83.83 | R14.A 16.51,83.83 | 16.51,83.83 20.32,83.83 | R5.A 20.32,83.83 | 20.32,83.83 24.13,83.83 | R12.A 24.13,83.83 | 24.13,83.83 27.94,83.83 | R11.A 27.94,83.83 | 27.94,83.83 31.75,83.83 | R10.A 31.75,83.83 | R9.A 35.56,83.83 | 35.56,81.93 35.56,83.83 | 35.56,83.83 33.34,83.83 | 31.75,83.83 33.34,83.83 | 33.34,83.83 v33.34,80.66 | IC3.10 60.33,70.5 v60.29,69.93
  Bottom 0.406: v70.48,93.67 70.48,102.25 69.85,102.88 | v33.34,80.66 33.34,64.78 | 60.39,65.1 60.71,64.78
  Bottom 1.016: 60.39,65.1 60.29,65.1 v60.29,69.93 | 51.44,102.25 50.8,102.88 | 2.54,65.42 1.91,64.78 | C23.+ 50.16,102.88
  Bottom 1.27: C22.+ 4.45,71.13 | C21.+ 4.45,96.53 | C19.+ 23.5,64.78 | C20.+ 15.24,64.78
  Bottom 2.54: 2.54,66.05 2.54,66.69 | 2.54,100.34 2.54,66.69 | 2.54,66.69 3.17,66.05 1.91,64.78 | 1.91,64.78 1.91,100.98 6.35,105.42 22.86,105.42 23.5,104.79 | 163.83,64.78 163.45,64.4 163.45,60.97 163.79,60.63 163.79,57.12 K2.1 158.88,51.96 161.93,48.91 161.93,24.27 K1.1 | 163.83,64.78 123.19,64.78 | 123.19,64.78 74.93,64.78 | 74.93,64.78 60.71,64.78 38.73,64.78 | 38.73,64.78 33.34,64.78 23.5,64.78 15.24,64.78 1.91,64.78 | 41.27,102.88 4.45,102.88 4.45,96.53 4.45,71.13 4.45,63.51 161.93,63.51 161.93,61.61 162.56,60.97 5.71,60.97 1.91,64.78 | 41.27,102.88 50.16,102.88 50.8,102.88 69.85,102.88 77.47,102.88 | 77.47,102.88 125.73,102.88 125.73,104.79 | 163.22,64.44 163.83,64.78 | 163.83,64.78 163.83,69.84 | K3.1 122.94,21.35 125.73,24.14 125.73,49.42 | 125.73,49.42 K4.1 | K5.1 74.55,21.22 77.47,24.14 77.47,49.16 K6.1 74.42,64.27 74.93,64.78 | K7.1 38.48,21.35 41.27,24.14 41.27,49.54 K8.1 38.61,64.66 38.73,64.78 | 125.73,49.42 125.73,49.54 123.19,52.08 123.19,64.78 | K12.1 125.73,151.14 125.73,125.74 | 125.73,125.74 125.73,125.62 K11.1 | K10.1 159.13,153.94 161.93,151.14 161.93,125.87 K9.1 | K14.1 74.68,153.94 77.47,151.14 77.47,125.87 K13.1 74.68,122.82 77.47,120.03 77.47,102.88 | K16.1 38.61,153.81 41.27,151.14 41.27,125.62 K15.1 41.27,120.03 41.27,102.88 | K9.1 159.13,122.82 | 125.73,125.74 123.19,123.2 123.19,122.57 125.73,120.03 | 125.73,120.03 125.73,104.79 | 8.26,104.79 23.5,104.79 | 23.5,104.79 125.73,104.79 | K9.1 158.88,121.42 157.48,120.03 125.73,120.03
N$4  (via drill 0.5)
  Top 0.254: IC1.15 v77.47,81.29 | RN1.3 114.45,96.04 115.57,97.17 115.57,98.44 116.2,99.07 118.75,99.07 JP1.A3
  Bottom 0.254: v77.47,81.29 75.56,81.29 74.93,81.93 74.93,99.07 76.2,100.34 119.38,100.34 120.02,99.71 JP1.A3
N$99
  Top 0.254: POWER1.A 173.6,38.23 173.23,37.86 171.95,37.86 RNB1.3
  Top 0.406: 171.91,37.99 RNB1.3
N$100
  Top 0.813: 139.06,73.8 IC6.8 147.5,73.8 H1.2 | 139.06,73.8 137.29,73.8 136.53,73.04 136.53,68.49 136.02,67.98 136.02,66.58 D1.C 135.87,66.43 133.86,66.43 132.97,67.32 125.73,67.32 124.84,68.21 CD1.2 | 139.04,73.82 139.06,73.8
N$101
  Top 0.813: CD1.1 127.15,74.79 128.27,73.67 133.1,73.67 133.22,73.8 IC6.1
N$405  (via drill 0.5)
  Top 0.229: IC1.21 85.09,78.43 84.45,77.8 71.12,77.8 70.48,78.43 IC3.1
  Top 0.254: 85.09,78.43 v85.09,80.78 | v99.31,77.99 99.95,77.36 102.01,77.36
  Top 0.305: 102.01,77.36 102.07,77.36 RN19.5
  Bottom 0.229: v85.09,80.78 85.09,80.66 85.72,81.29 98.68,81.29 99.31,80.66 v99.31,77.99
N$406  (via drill 0.5)
  Top 0.229: IC1.25 v90.18,77.74 90.17,75.89 89.53,75.26 66.04,75.26 65.41,75.89 IC3.5 | v95.89,73.99 99.38,73.99 99.69,73.67 102,73.67 RN18.5
  Bottom 0.229: v90.18,77.74 90.17,78.9 90.53,79.26 95.48,79.26 95.89,78.86 v95.89,73.99
N$407  (via drill 0.5)
  Top 0.229: IC1.26 v91.44,77.74 91.44,75.58 90.49,74.62 64.77,74.62 64.14,75.26 IC3.6 | v96.84,73.04 99.38,73.04 99.69,72.72 101.99,72.72 RN18.6
  Bottom 0.229: v91.44,77.74 91.44,78.63 91.57,78.75 94.74,78.75 94.87,78.63 94.87,73.29 95.12,73.04 v96.84,73.04
N$408  (via drill 0.5)
  Top 0.254: IC1.16 v78.74,82.56 | RN1.2 114.94,95.24 115.57,95.9 116.2,96.53 118.75,96.53 JP1.A2
  Bottom 0.254: v78.74,82.56 76.2,82.56 75.56,83.2 75.56,98.44 76.83,99.71 118.11,99.71 118.75,99.07 118.75,96.53 JP1.A2
N$409  (via drill 0.5)
  Top 0.229: IC1.22 86.36,77.8 85.72,77.17 69.85,77.17 69.22,77.8 IC3.2
  Top 0.254: 86.36,77.8 v86.36,77.74 | v98.3,77.23 99.06,77.23 99.69,76.59 102.05,76.59 RN19.6
  Bottom 0.229: v86.36,77.74 86.36,80.4 86.74,80.78 97.79,80.78 98.3,80.28 v98.3,77.23
N$410  (via drill 0.5)
  Top 0.229: IC1.23 87.63,77.17 87,76.53 68.58,76.53 67.94,77.17 IC3.3
  Top 0.254: 87.63,77.17 v87.63,77.74 | v97.41,76.21 98.93,76.21 99.31,75.83 102.05,75.83 RN19.7
  Bottom 0.229: v87.63,77.74 87.63,80.02 87.88,80.28 97.03,80.28 97.41,79.9 v97.41,76.21
  Bottom 0.254: 97.66,76.09 v97.41,76.21
N$411  (via drill 0.5)
  Top 0.229: IC1.24 88.9,76.53 88.27,75.89 67.31,75.89 66.67,76.53 IC3.4
  Top 0.254: 88.9,76.53 v88.9,77.74 | v97.03,74.94 102,74.94 RN19.8
  Bottom 0.229: v88.9,77.74 88.9,79.26 89.41,79.77 95.76,79.77 96.52,79.01 96.52,75.45 v97.03,74.94
N$416  (via drill 0.6)
  Top 0.203: 69.22,87.01 69.53,87.32 75.25,87.32 76.2,88.28 76.2,90.5 76.83,91.14 93.34,91.14 93.98,91.77 v93.98,96.53
  Top 0.229: v93.98,96.53 93.98,97.42 93.22,98.18 93.22,98.96 RN21.8
  Top 0.406: v93.98,90.18 IC1.1 | IC4.8 69.22,87.01
  Bottom 0.406: v93.98,96.53 v93.98,90.18
N$417  (via drill 0.6)
  Top 0.203: IC4.7 67.94,87.32 68.45,87.83 74.74,87.83 75.56,88.66 75.56,91.14 76.2,91.77 92.08,91.77 92.71,92.4 v92.71,96.53
  Top 0.229: v92.71,96.53 92.71,97.55 92.33,97.93 92.33,99.02 RN21.7
  Top 0.406: v92.71,90.18 IC1.2
  Bottom 0.406: v92.71,96.53 v92.71,90.18
N$418  (via drill 0.6)
  Top 0.203: IC4.6 66.67,87.64 67.37,88.34 73.98,88.34 74.93,89.29 74.93,91.77 75.56,92.4 90.81,92.4 91.44,93.04 v91.44,96.53
  Top 0.229: v91.44,96.53 91.44,98.06 91.57,98.18 91.57,99.02 RN21.6
  Top 0.406: v91.44,90.18 IC1.3
  Bottom 0.406: v91.44,96.53 v91.44,90.18
N$419  (via drill 0.6)
  Top 0.203: IC4.5 65.41,87.64 66.61,88.85 73.34,88.85 74.3,89.8 74.3,92.4 74.93,93.04 89.53,93.04 90.17,93.67 v90.17,96.53
  Top 0.229: v90.17,96.53 90.17,97.68 90.68,98.18 90.68,98.96 RN21.5
  Top 0.406: v90.17,90.18 IC1.4
  Bottom 0.406: v90.17,90.18 v90.17,96.53
N$420  (via drill 0.6)
  Top 0.203: IC4.4 64.14,87.64 65.85,89.36 72.83,89.36 73.66,90.18 73.66,93.04 74.3,93.67 88.27,93.67 88.9,94.31 v88.9,96.53
  Top 0.229: v88.9,96.53 88.9,97.29 88.27,97.93 88.27,98.96 RN20.8
  Top 0.406: v88.9,90.18 IC1.5
  Bottom 0.406: v88.9,96.53 v88.9,90.18
N$421  (via drill 0.6)
  Top 0.203: IC4.3 62.87,87.64 65.09,89.87 72.33,89.87 73.03,90.56 73.03,93.67 73.66,94.31 87,94.31 87.63,94.95 v87.63,96.53
  Top 0.229: v87.63,96.53 87.63,97.68 87.38,97.93 87.38,99.02 RN20.7
  Top 0.406: v87.63,90.18 IC1.6
  Bottom 0.406: v87.63,96.53 v87.63,90.18
N$422  (via drill 0.6)
  Top 0.203: IC4.2 61.59,87.64 64.33,90.37 71.69,90.37 72.39,91.07 72.39,94.31 73.03,94.95 85.91,94.95 86.36,95.39 v86.36,96.53
  Top 0.229: IC1.7 86.36,88.28 | v86.36,96.53 86.36,97.55 86.61,97.8 86.61,99.02 RN20.6
  Top 0.406: 86.36,96.16 v86.36,96.53 | v86.36,90.18 IC1.7
  Bottom 0.406: v86.36,96.53 v86.36,90.18
N$423  (via drill 0.6)
  Top 0.203: IC4.1 60.33,87.64 63.69,91.01 71.18,91.01 71.75,91.58 71.75,94.87 72.47,95.58 84.64,95.58 85.09,96.03 v85.09,96.53
  Top 0.229: v85.09,96.53 85.09,97.55 85.72,98.18 85.72,98.96 RN20.5
  Top 0.406: v85.09,90.18 IC1.8
  Bottom 0.406: v85.09,90.18 v85.09,96.53
N$441
  Top 0.406: RN5.1 40.71,91.38 40.01,92.09 13.86,92.09 R16.C
N$442
  Top 0.406: RN8.7 RN7.2
N$443
  Top 0.406: RN7.3 RN8.6
N$444
  Top 0.406: RN8.5 RN7.4
N$445
  Top 0.406: RN5.2 40.24,90.58 39.37,91.45 17.03,91.45 R15.C
N$447
  Top 0.406: RN5.4 39.3,88.98 38.1,90.18 23.38,90.18 R13.C
N$448
  Top 0.406: RN5.5 RN6.4
N$449
  Top 0.406: RN7.1 RN8.8
N$450
  Top 0.406: RN8.1 39.44,87.57 37.47,89.55 26.55,89.55 R12.C
N$451
  Top 0.406: RN5.6 RN6.3
N$452
  Top 0.406: RN8.2 38.97,86.77 36.83,88.91 29.73,88.91 R11.C
N$453
  Top 0.406: RN6.2 RN5.7
N$454
  Top 0.406: RN5.8 RN6.1
N$458
  Top 0.406: RN5.3 39.77,89.78 38.73,90.82 20.2,90.82 R14.C
N$459
  Top 0.406: RN8.3 38.5,85.97 36.2,88.28 32.91,88.28 R10.C
N$463
  Top 0.406: RN12.4 RN11.5
N$470
  Top 0.406: RN8.4 38.03,85.17 36.2,87.01 35.67,87.01 R9.C
N$473
  Top 0.406: RN12.5 38.03,82.49 36.2,80.66 35.67,80.66 R1.C
N$474
  Top 0.406: RN11.6 RN12.3
N$475
  Top 0.406: RN12.6 38.5,81.69 36.2,79.39 32.91,79.39 R2.C
N$476
  Top 0.406: RN12.7 38.97,80.89 36.83,78.75 29.73,78.75 R3.C
N$477
  Top 0.406: RN9.4 RN10.5
N$478
  Top 0.406: RN10.6 RN9.3
N$479
  Top 0.406: RN9.2 RN10.7
N$480
  Top 0.406: RN10.8 RN9.1
N$481
  Top 0.406: RN12.2 RN11.7
N$482
  Top 0.406: RN10.1 39.3,78.68 38.1,77.48 23.38,77.48 R5.C
N$483
  Top 0.406: RN12.8 39.44,80.09 37.47,78.12 26.55,78.12 R4.C
N$484
  Top 0.406: RN10.3 40.24,77.08 39.37,76.21 17.03,76.21 R7.C
N$485
  Top 0.406: RN10.4 40.71,76.28 40.01,75.58 13.86,75.58 R8.C
N$486
  Top 0.406: RN10.2 39.77,77.88 38.73,76.85 20.2,76.85 R6.C
N$498  (via drill 0.5)
  Top 0.254: IC1.17 80.01,83.2 v79.38,83.83 | RN1.1 115.75,94.44 116.2,93.99 118.75,93.99 JP1.A1
  Bottom 0.254: v79.38,83.83 76.83,83.83 76.2,84.47 76.2,97.8 77.47,99.07 115.57,99.07 116.2,98.44 116.2,92.09 116.84,91.45 118.75,91.45 JP1.A1
N$500
  Top 0.406: RN11.8 RN12.1
N$524
  Bottom 2.54: 164.47,69.86 163.83,69.86
N$525  (via drill 0.5)
  Top 0.229: IC3.7 62.87,74.62 63.5,73.99 91.76,73.99 92.71,74.94 v92.71,77.74 IC1.27 | v97.79,72.09 101.52,72.09 RN18.7
  Bottom 0.229: v97.79,72.09 93.03,72.09 92.71,72.4 v92.71,77.74
N$526
  Top 0.229: IC1.28 93.98,73.99 | 93.98,73.99 93.34,73.36 62.23,73.36 61.59,73.99 IC3.8 | 93.98,73.99 93.98,71.77 94.61,71.13 102,71.13 RN18.8
OC_R1_A  (via drill 0.6)
  Top 0.406: IC3.18 v70.48,69.93 70.48,68.59 71.12,67.96 123.19,67.96 128.27,62.88 128.27,47 130.18,45.1 159.38,45.1 161.29,43.19 161.29,13.47 K1.2 | RN11.4 58.35,82.49 v58.55,82.31
  Bottom 0.406: v58.55,82.31 70.1,82.31 70.48,81.93 v70.48,69.93
OC_R1_B
  Top 0.203: RN7.5 57.22,85.17 63.82,91.77 68.26,91.77 69.22,92.72 IC4.11
  Top 0.406: IC4.11 69.22,100.34 69.85,100.98 80.64,100.98 81.28,101.61 124.83,101.61 125.73,102.51 125.73,119.39 126.36,120.03 156.84,120.03 158.75,118.12 158.75,112.53 K9.2
OC_R2_A  (via drill 0.6)
  Top 0.406: RN11.3 56.75,81.69 v57.15,81.29 | IC3.17 v69.22,69.93 69.22,67.32 69.85,66.69 122.56,66.69 127,62.24 127,46.37 129.54,43.83 156.84,43.83 158.62,42.05 K2.2
  Bottom 0.406: v57.15,81.29 67.94,81.29 69.22,80.02 v69.22,69.93
OC_R2_B
  Top 0.203: IC4.12 67.94,93.36 66.99,92.4 63.82,92.4 57.38,85.97 RN7.6
  Top 0.406: IC4.12 67.94,100.98 68.58,101.61 80.01,101.61 80.64,102.25 124.2,102.25 125.09,103.15 125.09,119.76 125.99,120.66 156.21,120.66 156.84,121.3 156.84,141.74 K10.2
OC_R3_A  (via drill 0.6)
  Top 0.406: RN11.2 55.01,80.89 v55.88,80.02 | IC3.16 v67.94,69.93 67.94,66.69 69.22,65.42 121.28,65.42 125.73,60.97 125.73,13.98 122.94,11.19 K3.2
  Bottom 0.406: v55.88,80.02 66.67,80.02 67.94,78.75 v67.94,69.93
OC_R3_B
  Top 0.203: RN7.7 57.55,86.77 63.82,93.04 66.36,93.04 66.67,93.36 IC4.13
  Top 0.406: IC4.13 66.67,101.61 67.31,102.25 79.38,102.25 80.01,102.88 121.92,102.88 122.56,103.52 122.56,112.28 K11.2
OC_R4_A  (via drill 0.6)
  Top 0.406: RN11.1 53.27,80.09 v54.61,78.75 | IC3.15 v66.67,69.93 66.67,66.05 68.58,64.15 119.38,64.15 120.65,62.88 120.65,44.46 122.94,42.18 K4.2
  Bottom 0.406: v54.61,78.75 65.41,78.75 66.67,77.48 v66.67,69.93
OC_R4_B
  Top 0.203: RN7.8 57.72,87.57 63.82,93.67 65.09,93.67 65.41,93.99 IC4.14
  Top 0.406: IC4.14 65.41,102.25 66.04,102.88 78.74,102.88 79.44,103.58 120.02,103.58 120.9,104.47 120.9,141.74 K12.2
OC_R5_A  (via drill 0.6)
  Top 0.406: RN9.8 52.14,78.68 53.34,77.48 v58.42,77.48 | IC3.14 v65.41,69.93 65.41,65.73 77.47,53.67 77.47,14.11 K5.2
  Bottom 0.406: v58.42,77.48 64.14,77.48 65.41,76.21 v65.41,69.93
OC_R5_B
  Top 0.203: IC4.15 64.14,94.63 63.82,94.31 63.5,94.31 58.17,88.98 RN6.5
  Top 0.406: IC4.15 64.14,102.88 64.77,103.52 73.03,103.52 74.55,105.04 74.55,112.53 K13.2
OC_R6_A  (via drill 0.6)
  Top 0.406: RN9.7 51.67,77.88 53.34,76.21 v57.15,76.21 | IC3.13 v64.14,69.93 64.14,65.42 72.39,57.16 72.39,44.08 K6.2
  Bottom 0.406: v57.15,76.21 62.87,76.21 64.14,74.94 v64.14,69.93
OC_R6_B
  Top 0.203: RN6.6 58.02,89.78 62.87,94.63 IC4.16
  Top 0.406: IC4.16 62.87,103.52 64.14,104.79 70.48,104.79 72.39,106.69 72.39,141.74 K14.2
OC_R7_A  (via drill 0.6)
  Top 0.406: RN9.6 51.2,77.08 53.34,74.94 v55.88,74.94 | IC3.12 v62.87,69.93 62.87,67.32 62.23,66.69 42.55,66.69 41.27,65.42 41.27,13.35 38.99,11.06 K7.2
  Bottom 0.406: v55.88,74.94 61.59,74.94 62.87,73.67 v62.87,69.93
OC_R7_B
  Top 0.203: RN6.7 57.87,90.58 61.59,94.31 IC4.17
  Top 0.406: IC4.17 61.59,101.61 60.96,102.25 38.73,102.25 38.35,102.63 38.35,112.53 K15.2
OC_R8_A  (via drill 0.6)
  Top 0.406: RN9.5 50.73,76.28 53.34,73.67 v54.61,73.67 | IC3.11 v61.59,69.93 61.59,68.59 60.96,67.96 36.83,67.96 35.56,66.69 35.56,45.1 K8.2
  Bottom 0.406: v54.61,73.67 60.33,73.67 61.59,72.4 v61.59,69.93
OC_R8_B
  Top 0.203: RN6.8 57.72,91.38 60.33,93.99 IC4.18
  Top 0.406: IC4.18 60.33,100.98 59.69,101.61 37.15,101.61 36.45,102.31 36.45,141.62 K16.2
REG_5V  (via drill 0.5, 0.6, 0.9)
  Top 0.254: 170.22,37.99 169.04,37.99 v168.28,38.75 | RN3.6 RN3.5 148.21,92.32 148.21,92.85 147.83,93.23 v147.83,93.61
  Top 0.305: 81.28,85.1 82.55,86.37 83.19,86.37 83.82,87.01 | IC1.18 v81.28,84.47 | IC1.9 83.82,87.01 | 83.82,87.01 84.45,86.37 94.93,86.37 95.25,86.37 | 170.22,37.99 RNB1.6
  Top 0.61: v147.83,93.61 149.61,93.61 153.03,90.18 X10.2
  Top 0.813: H1.1 142.72,67.8 v142.24,67.32 | IC6.4 133.48,69.99 | 133.48,69.99 v133.35,69.86 | 133.48,69.99 130.41,69.99 C10.1
  Top 1.016: C25.+ 107.31,77.74 106.55,78.5 102.49,78.5 101.69,79.3 C1.1 C4.1 101.69,86.92 | C6.1 96.29,85.33 95.25,86.37 | C6.1 C7.1 | 101.69,86.92 100.97,87.64 100.33,87.64 | 100.33,87.64 97.16,87.64 96.52,87.01 96.52,85.33 C6.1 | 101.69,86.92 101.69,87.09 102.87,88.28 C27.+ 110.49,90.82 112.39,92.72 JP1.B1 | C26.+ 100.33,87.64
  Top 1.27: 94.93,86.37 84.14,86.37 83.82,86.69 82.87,86.69 81.28,85.1 v81.28,84.47 | H1.1 151.23,66.53 v151.76,66.94
  Bottom 0.254: JP1.B3 JP1.B2 JP1.B1 | v168.28,38.75 168.28,50.18 169.54,51.45 173.99,51.45 175.26,52.72 175.26,74.31 175.9,74.94 175.9,89.55 175.26,90.18 v170.56,90.18
  Bottom 0.61: FOR_NANO.5V 146.05,95.39 | 146.05,95.39 v147.83,93.61 | 146.05,95.39 146.05,95.26 145.41,94.63 133.99,94.63 132.72,93.36 | v131.44,93.36 128.91,93.36 125.73,90.18 112.39,90.18 C27.+
  Bottom 0.813: v142.24,67.32 133.35,67.32 v133.35,69.86 132.08,71.13 132.08,81.93 133.35,83.2 133.35,92.72 132.72,93.36 v131.44,93.36
  Bottom 1.016: v170.56,90.18 X10.2
  Bottom 1.27: C24.+ v81.28,84.47
REG_12V  (via drill 0.5)
  Top 0.813: BRA2.+ 158.12,71.13 156.21,68.59 148.59,68.59 144.78,72.4 142.49,72.4 v138.3,72.53 IC6.7 | C9.1 130.3,82.44 131.44,81.29 132.72,81.29 133.35,80.66 v133.35,75.58
  Bottom 0.813: v133.35,75.58 133.35,73.67 134.49,72.53 v138.3,72.53
UNREG_12V
  Top 2.54: 162.51,66.05 BRA2.~@1 BRA2.~@2 | 162.51,66.05 U$6.TIP | 162.51,66.05 162.51,61.27 163.45,60.34 173.03,60.34 X17.2

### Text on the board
tNames: Bank 2 | 8 | 6 | 4 | 2 | 7 | 5 | 3 | 1 | MCP23017 | ANSR16x0 | REV.A | Address: | A0 | A1 | 2016 ControlEverything.com | GND | A2 | +5V | SC | SDA | SCL | 12V DC / Power / Supply | 12V DC / Power / Supply | 12V DC / Power / Supply | 8 | 6 | 4 | 2 | 7 | 5 | 3 | 1 | Bank 1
